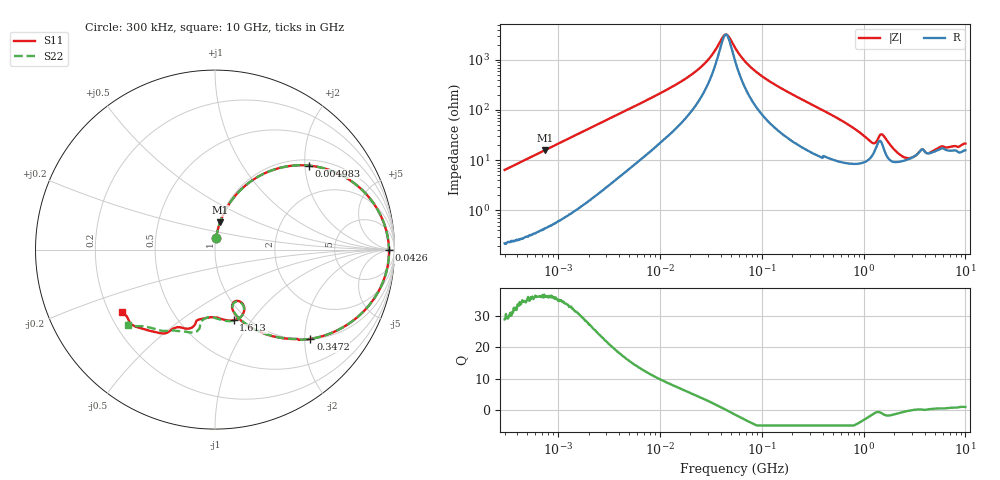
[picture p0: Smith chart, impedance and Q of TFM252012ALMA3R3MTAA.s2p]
! S-Parameter Data Generated by TDK Corporation
! Copyright(C) 2019 TDK Corporation.
! All Rights Reserved.
! TDK P/N: TFM252012ALMA3R3MTAA (Inductor)
! Property: L=3.3uH at 1MHz
! Size(LxWxT): 2.5x2x1.2mm
! Model Type: s2p (Touchstone File Format Version 1.0)
! Frequency: DC=Yes Start=0.3MHz Stop=10000MHz 802points Log-sweep
! Model Generated on May 10, 2019
! Port Assignments:
!  1 ---@@@--- 2
! Applicable Conditions:
!  Temperature = 25 degC
!  DC Bias Current = 0 A
!  Small Signal Operation
! Terms and conditions regarding TDK Simulation Models
! (1)This simulation model is being provided solely for informational purposes. Please refer to the specifications of the products in terms of detailed characteristics of such products.
! (2)In no event shall TDK Corporation of any of its subsidiaries be liable for any loss or damage arising, directly or indirectly,
!  From any information contained in this simulation model, including, but not limited to loss or damages arising from any inaccuracies, omissions or errors in connection with such information.
! (3)Any and all copyrights on this simulation model are owned by TDK Corporation.
!  Duplication or redistribution of this simulation model without prior written permission from TDK Corporation is prohibited.
! (4)This simulation model is subject to any modification or change without any prior notice.
! (5)Neither TDK Corporation nor any of its subsidiaries shall make any warranty, express or implied,
!  Including but not limited to the correctness, implied warranties of merchantability and fitness for a particular purpose with respect to this simulation models.
! (6)The use of this simulation model shall be deemed to have consented to the terms and conditions hereof.
# Hz S MA R 50
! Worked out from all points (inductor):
!   801 points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, 300 kHz to 10 GHz, reference 50 ohm
!   read as one part in series: L = 3.39 uH near 318.3 kHz
!   highest Q = 36.3 at 742.2 kHz (marker M1), where L = 3.38 uH
!   self-resonance near 44.6 MHz
!   S11 on the Smith chart (normalised r, x): 300 kHz: 1.00, +0.13; 4.983 MHz: 1.14, +2.09; 42.6 MHz: 64, -4; 347.2 MHz: 1.01, -2.13; 1.613 GHz: 0.87, -0.82; 10 GHz: 0.25, -0.29
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300000  0.06381 84.5  0.9957 -3.7  0.9956 -3.6  0.06394 84.4
742172  0.1552 79.5  0.9836 -8.9  0.9835 -8.9  0.1552 79.5
1713600  0.337 68.4  0.9303 -19.7  0.9302 -19.7  0.3369 68.4
4982740  0.7004 41.9  0.6706 -44.4  0.6706 -44.4  0.7003 41.9
9671944  0.866 24.6  0.4214 -59.7  0.4214 -59.7  0.866 24.6
2.473055e7  0.9573 7.4  0.1399 -68.7  0.1399 -68.8  0.9573 7.4
3.206042e7  0.9655 3.7  0.08069 -63.1  0.0807 -63.1  0.9656 3.8
4.259986e7  0.9693 -0.1  0.03213 -18.6  0.03216 -18.6  0.9696 -0.1
4.68602e7  0.9695 -1.4  0.03226 18.7  0.03228 18.7  0.9697 -1.3
5.477226e7  0.9684 -3.6  0.05529 53.2  0.0553 53.2  0.9687 -3.5
7.58404e7  0.9605 -8.3  0.1272 67.3  0.1272 67.3  0.9609 -8.2
1.050124e8  0.9427 -13.8  0.2117 66.8  0.2117 66.8  0.9433 -13.6
3.126428e8  0.7586 -39.9  0.5752 44.0  0.5752 44.0  0.76 -39.8
3.471693e8  0.7281 -43.1  0.6117 40.9  0.6117 40.9  0.7296 -42.9
8.758105e8  0.4225 -69.7  0.8347 10.9  0.8347 10.9  0.4242 -69.3
1.292013e9  0.3094 -69.4  0.8249 -4.2  0.8248 -4.3  0.3132 -69.2
1.613252e9  0.4073 -75.2  0.7924 -3.2  0.7924 -3.2  0.41 -76.0
1.767019e9  0.3947 -82.3  0.8262 -6.2  0.8262 -6.2  0.3965 -83.4
2.446702e9  0.3778 -93.9  0.836 -18.4  0.8359 -18.4  0.3782 -95.5
3.472057e9  0.4092 -104.5  0.7801 -32.3  0.7801 -32.3  0.4181 -101.3
6.41458e9  0.5568 -123.2  0.6539 -55.1  0.654 -55.1  0.5489 -125.8
1e10  0.6239 -146.0  0.5392 -79.1  0.5393 -79.2  0.6432 -139.1
